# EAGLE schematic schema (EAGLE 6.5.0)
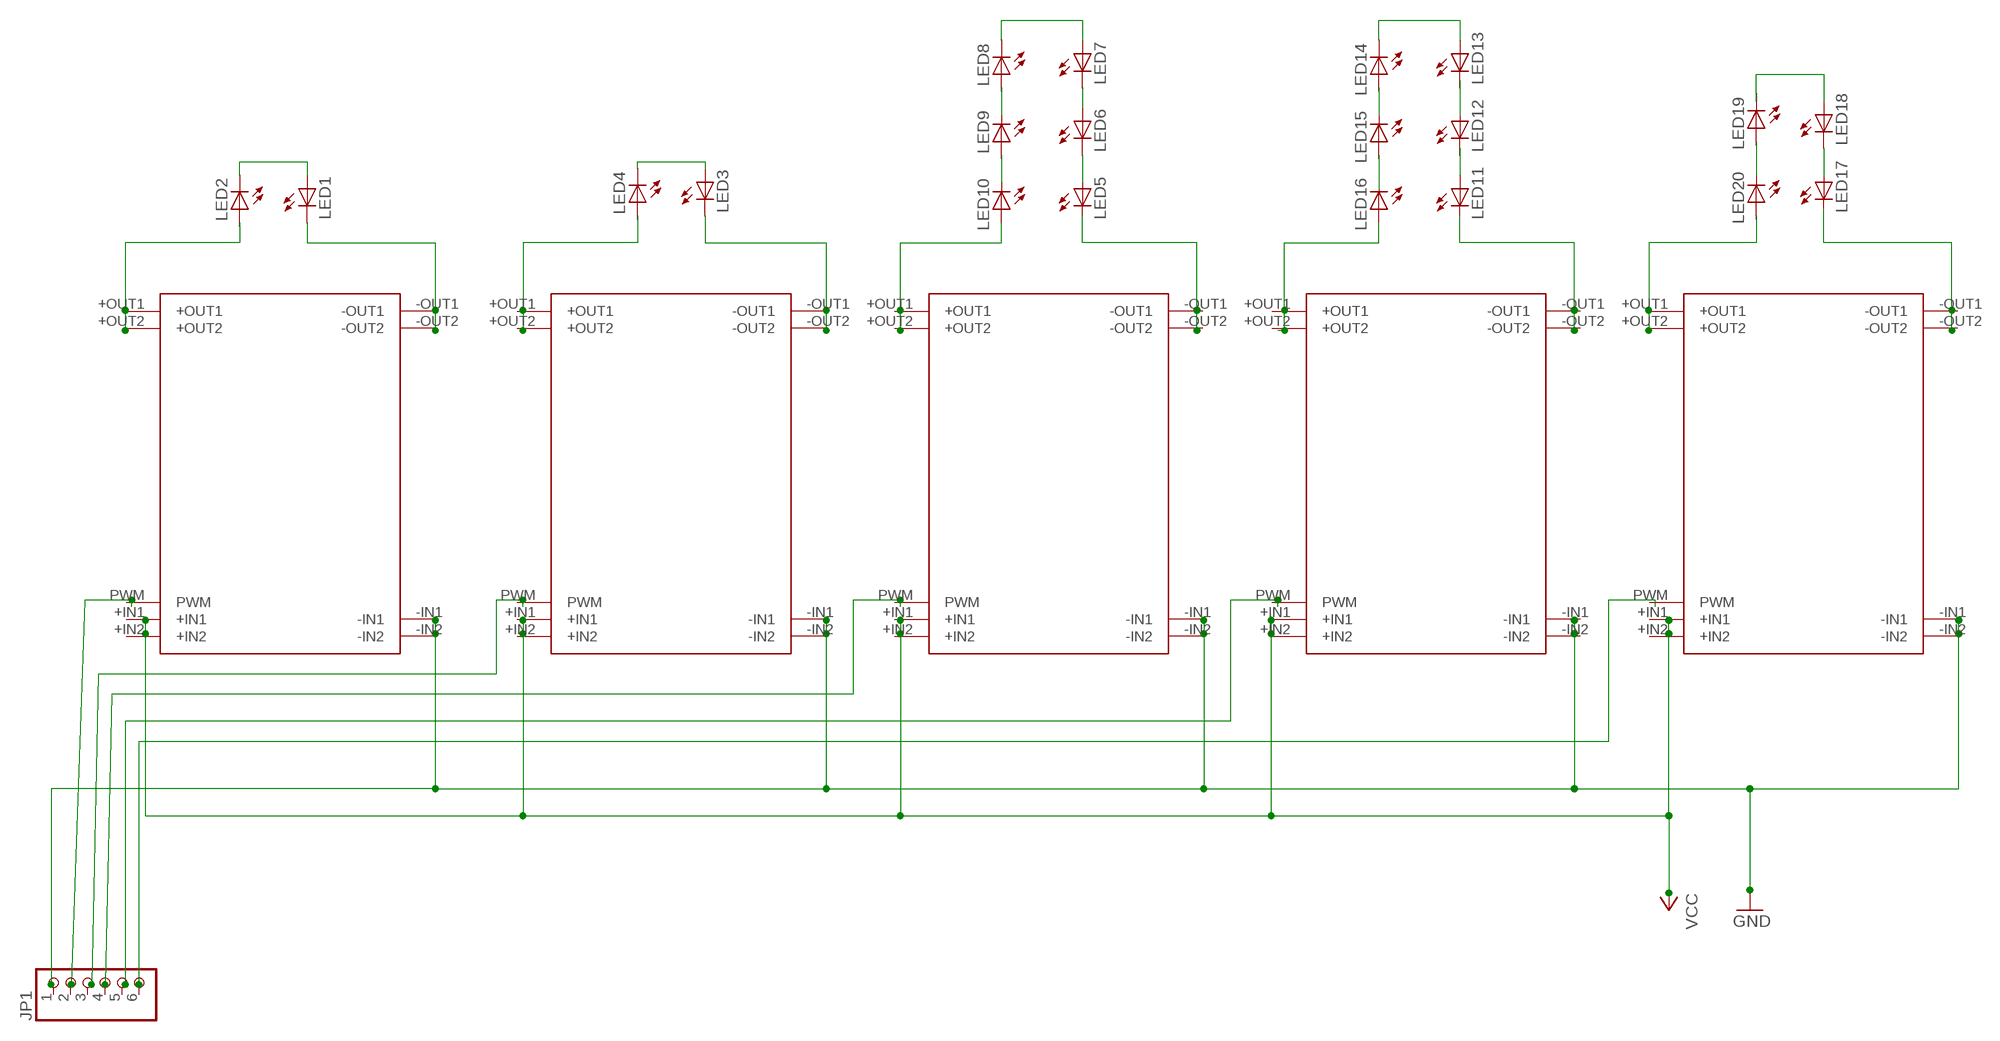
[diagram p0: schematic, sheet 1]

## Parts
JP1  PINHD-1X6CLEAN  [1X06-CLEAN]
LED1  LED-LUMILED+  [LUMILED+]
LED2  LED-LUMILED+  [LUMILED+]
LED3  LED-LUMILED+  [LUMILED+]
LED4  LED-LUMILED+  [LUMILED+]
LED5  LED-LUMILED+  [LUMILED+]
LED6  LED-LUMILED+  [LUMILED+]
LED7  LED-LUMILED+  [LUMILED+]
LED8  LED-LUMILED+  [LUMILED+]
LED9  LED-LUMILED+  [LUMILED+]
LED10  LED-LUMILED+  [LUMILED+]
LED11  LED-LUMILED+  [LUMILED+]
LED12  LED-LUMILED+  [LUMILED+]
LED13  LED-LUMILED+  [LUMILED+]
LED14  LED-LUMILED+  [LUMILED+]
LED15  LED-LUMILED+  [LUMILED+]
LED16  LED-LUMILED+  [LUMILED+]
LED17  LED-LUMILED+  [LUMILED+]
LED18  LED-LUMILED+  [LUMILED+]
LED19  LED-LUMILED+  [LUMILED+]
LED20  LED-LUMILED+  [LUMILED+]
U$1  LDD-H  [LDD]
U$2  LDD-H  [LDD]
U$3  LDD-H  [LDD]
U$4  LDD-H  [LDD]
U$6  LDD-H  [LDD]
Unconnected: JP1.1 JP1.2 JP1.3 JP1.4 JP1.5 JP1.6 LED1.2+(A) LED1.4-(C) LED2.2+(A) LED2.4-(C) LED3.2+(A) LED3.4-(C) LED4.2+(A) LED4.4-(C) LED5.2+(A) LED5.4-(C) LED6.2+(A) LED6.4-(C) LED7.2+(A) LED7.4-(C) LED8.2+(A) LED8.4-(C) LED9.2+(A) LED9.4-(C) LED10.2+(A) LED10.4-(C) LED11.2+(A) LED11.4-(C) LED12.2+(A) LED12.4-(C) LED13.2+(A) LED13.4-(C) LED14.2+(A) LED14.4-(C) LED15.2+(A) LED15.4-(C) LED16.2+(A) LED16.4-(C) LED17.2+(A) LED17.4-(C) LED18.2+(A) LED18.4-(C) LED19.2+(A) LED19.4-(C) LED20.2+(A) LED20.4-(C) U$1.+IN1 U$1.+IN2 U$1.+OUT1 U$1.+OUT2 U$1.-IN1 U$1.-IN2 U$1.-OUT1 U$1.-OUT2 U$1.PWM U$2.+IN1 U$2.+IN2 U$2.+OUT1 U$2.+OUT2 U$2.-IN1 U$2.-IN2 U$2.-OUT1 U$2.-OUT2 U$2.PWM U$3.+IN1 U$3.+IN2 U$3.+OUT1 U$3.+OUT2 U$3.-IN1 U$3.-IN2 U$3.-OUT1 U$3.-OUT2 U$3.PWM U$4.+IN1 U$4.+IN2 U$4.+OUT1 U$4.+OUT2 U$4.-IN1 U$4.-IN2 U$4.-OUT1 U$4.-OUT2 U$4.PWM U$6.+IN1 U$6.+IN2 U$6.+OUT1 U$6.+OUT2 U$6.-IN1 U$6.-IN2 U$6.-OUT1 U$6.-OUT2 U$6.PWM

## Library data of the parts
JP1 = adafruit:PINHD-1X6: PIN HEADER
LED1-LED20 = led:LED: LED
U$1-U$4 U$6 = ldd:LDD-H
